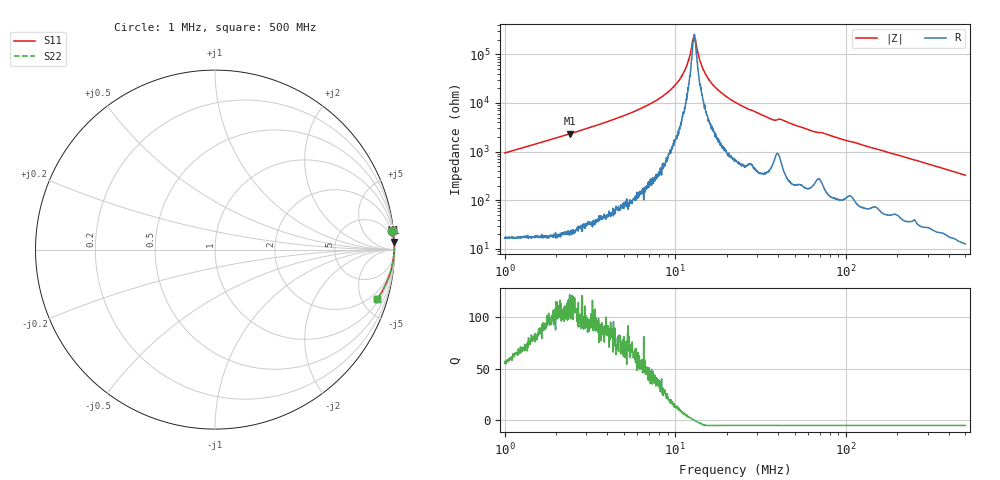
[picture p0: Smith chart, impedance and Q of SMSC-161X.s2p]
!s-Parameter Generated by FASTRON Sdn. Bhd.
!FASTRON P/N : SMSC-161X
!Keysight Technologies,E4991B,MY54100416,A.01.15
!Date: Thu Mar 19 14:28:49 2026
!Version  : Rev00 Thu Mar 19 14:28:49 2026
!Data & Calibration Information:
!PortZ  Port1:50+j0  Port2:50+j0
!When reading, reference impedance value at option line is always used.
! Remarks : This data is being provided solely for informational purposes.
!Freq	S11	S21	S12	S22
# Hz S dB R 50
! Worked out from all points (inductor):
!   1601 points, 1 MHz to 500 MHz, reference 50 ohm
!   read as one part in series: L = 148 uH near 1.032 MHz
!   highest Q = 113 at 2.415 MHz (marker M1), where L = 153 uH
!   self-resonance near 12.88 MHz
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1000000  -0.07 6.1  -19.49 -82.9  -19.49 -82.9  -0.07 6.1
2414996  -0.01 2.5  -27.35 -87.1  -27.35 -87.1  -0.01 2.5
2820919  -0.01 2.1  -28.82 -87.4  -28.82 -87.4  -0.01 2.1
5396294  -0.00 0.9  -35.71 -88.1  -35.71 -88.1  -0.00 0.9
7957584  -0.00 0.5  -41.64 -87.9  -41.64 -87.9  -0.00 0.5
9440672  -0.00 0.3  -45.60 -86.8  -45.60 -86.8  -0.00 0.3
1.081541e7  -0.00 0.2  -50.60 -83.8  -50.60 -83.8  -0.00 0.2
1.168907e7  -0.00 0.1  -55.39 -74.5  -55.39 -74.5  -0.00 0.1
1.210491e7  -0.00 0.1  -59.04 -68.8  -59.04 -68.8  -0.00 0.1
1.263331e7  -0.00 0.0  -65.46 -41.9  -65.46 -41.9  -0.00 0.0
1.293118e7  -0.00 -0.0  -68.18 8.8  -68.18 8.8  -0.00 -0.0
1.318477e7  -0.00 -0.0  -64.95 40.5  -64.95 40.5  -0.00 -0.0
1.37603e7  -0.00 -0.1  -58.73 66.9  -58.73 66.9  -0.00 -0.1
1.419459e7  -0.00 -0.1  -55.78 73.7  -55.78 73.7  -0.00 -0.1
1.558143e7  -0.00 -0.2  -50.07 82.2  -50.07 82.2  -0.00 -0.2
1.798958e7  -0.00 -0.3  -45.01 84.6  -45.01 84.6  -0.00 -0.3
2.236068e7  -0.01 -0.5  -40.37 85.7  -40.37 85.7  -0.01 -0.5
3.690536e7  -0.02 -1.2  -33.21 82.3  -33.21 82.3  -0.02 -1.2
4.178966e7  -0.03 -1.2  -33.21 81.6  -33.21 81.6  -0.03 -1.2
6.307767e7  -0.03 -2.1  -28.52 83.8  -28.52 83.8  -0.03 -2.1
1.77937e8  -0.09 -6.0  -19.67 81.1  -19.67 81.1  -0.09 -6.0
5e8  -0.48 -16.9  -10.75 70.9  -10.75 70.9  -0.48 -16.9
